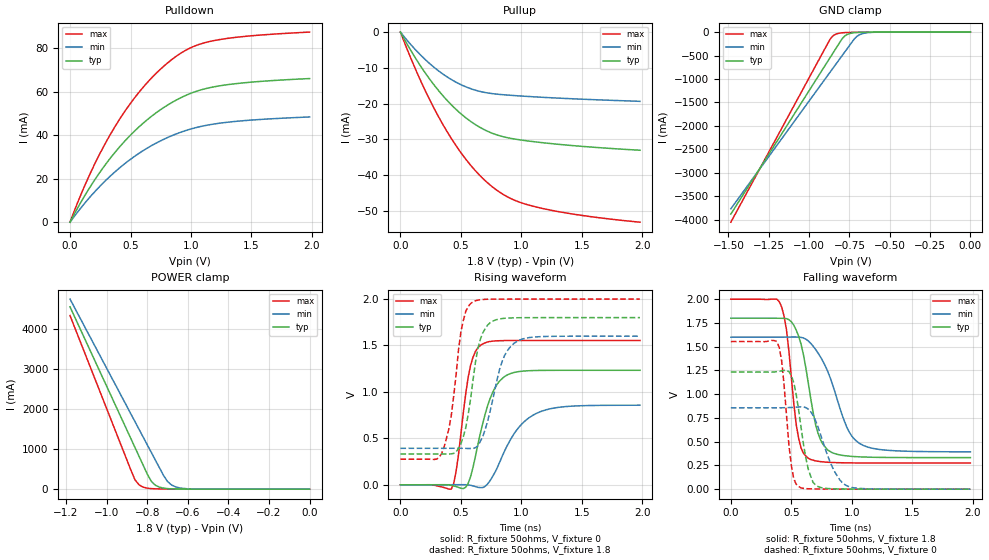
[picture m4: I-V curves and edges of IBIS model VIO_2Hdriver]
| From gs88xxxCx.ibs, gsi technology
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|  signals   DQA1-DQA9, DQB1-DQB9, DQC1-DQC9, DQD1-DQD9
[Model]   VIO_2Hdriver
Model_type   I/O
Polarity   Non-Inverting
Vinl  =   0.80v
Vinh  =   1.20v
Vmeas =   0.90v
Cref  =   0.0pF
Rref  =   50
Vref  =   0.90v
|  variable   typ   min   max
C_comp   3.0pF   2.5pF   3.5pF
|  variable   typ   min   max
[Temperature Range]   50   0   100
|  variable   typ   min   max
[Voltage Range]   1.8   1.6   2.0
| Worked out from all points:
|   slope of the pulldown table from 0 to 0.27 V, typ, clamps not added: 10.9 ohm
|   slope of the pullup table from 0 to 0.27 V, typ, clamps not added: 18.7 ohm
|   GND clamp passes 1 mA (typ) near -0.61 V on its own axis
|   POWER clamp passes 1 mA (typ) near -0.59 V on its own axis
|   rising waveform, R_fixture 50ohms, V_fixture 0: 20-80 % time 150ps typ, 233ps min, 94.8ps max; typ from 0 V to 1.23 V
|   rising waveform, R_fixture 50ohms, V_fixture 1.8: 20-80 % time 106ps typ, 141ps min, 98.2ps max; typ from 0.332 V to 1.8 V
|   falling waveform, R_fixture 50ohms, V_fixture 1.8: 20-80 % time 128ps typ, 210ps min, 86.5ps max; typ from 1.8 V to 0.332 V
|   falling waveform, R_fixture 50ohms, V_fixture 0: 20-80 % time 92.3ps typ, 153ps min, 65.9ps max; typ from 1.23 V to 0 V
[Pulldown]
| voltage   typ   min   max
0V        -286.4pA   -891.3pA   -166.8pA
80mV      8.2mA      5.874mA    11.32mA
180mV     17.4mA     12.49mA    23.94mA
280mV     25.51mA    18.36mA    35mA
380mV     32.65mA    23.54mA    44.68mA
480mV     38.89mA    28.08mA    53.1mA
600mV     45.29mA    32.74mA    61.72mA
820mV     54.3mA     39.26mA    73.82mA
1V        59.29mA    42.86mA    80.26mA
1.18V     62.12mA    45.04mA    83.37mA
1.48V     64.3mA     46.86mA    85.59mA
1.98V     66.03mA    48.39mA    87.39mA
[Pullup]
| voltage (VDDQ-Vout)   typ   min   max
0V        191.8pA    794.2pA    89.01pA
80mV      -4.802mA   -3.277mA   -6.819mA
180mV     -10.18mA   -6.867mA   -14.56mA
280mV     -14.87mA   -9.905mA   -21.45mA
380mV     -18.89mA   -12.4mA    -27.52mA
560mV     -24.48mA   -15.57mA   -36.39mA
660mV     -26.69mA   -16.61mA   -40.22mA
760mV     -28.3mA    -17.21mA   -43.28mA
920mV     -29.76mA   -17.7mA    -46.67mA
1.12V     -30.72mA   -18.13mA   -48.9mA
1.48V     -31.9mA    -18.73mA   -51.17mA
1.98V     -33.04mA   -19.37mA   -53.16mA
[GND Clamp]
| voltage   typ   min   max
-1.485V   -3.884A    -3.771A    -4.056A
-885mV    -626.9mA   -926.9mA   -247.2mA
-870mV    -545.6mA   -856mA     -153.5mA
-855mV    -464.4mA   -785mA     -89.11mA
-825mV    -301.9mA   -643.2mA   -32.88mA
-795mV    -141.5mA   -501.4mA   -15.38mA
-780mV    -86.61mA   -430.5mA   -11.65mA
-750mV    -32.85mA   -288.8mA   -7.734mA
-705mV    -8.727mA   -95.28mA   -4.834mA
-660mV    -2.907mA   -24.97mA   -2.925mA
-555mV    -316.7uA   -1.176mA   -484.9uA
0V        -278.2pA   -874.6pA   -161.2pA
[POWER Clamp]
| voltage (VDDQ-Vout)   typ   min   max
-1.18V    4.545A     4.74A      4.328A
-880mV    1.258A     1.875A     474.1mA
-860mV    1.039A     1.684A     234.3mA
-840mV    820.4mA    1.493A     107.4mA
-820mV    601.5mA    1.302A     50.64mA
-780mV    197.3mA    920.5mA    14.28mA
-760mV    99.71mA    729.7mA    9.034mA
-720mV    26.23mA    348.2mA    4.898mA
-700mV    13.96mA    192.6mA    3.916mA
-660mV    4.495mA    57.55mA    2.579mA
-560mV    510.5uA    2.941mA    648.3uA
0V        209pA      794.1pA    88.9pA
[Ramp]
| voltage   typ   min   max
dV/dt_r   1.16/125p   1.0/182p   1.35/88p
dV/dt_f   1.25/134p   1.12/205p   1.40/91p
R_load  =   50ohms
[Rising Waveform]
C_fixture =   0.0pF
R_fixture =   50ohms
V_fixture =   0
| Time   V(typ)   V(min)   V(max)
0s        2.247nV    9.209nV    987.5pV
420ps     -6.194mV   384.6uV    -47.41mV
460ps     -19.49mV   604.6uV    143.7mV
540ps     -26.68mV   586.1uV    982.9mV
580ps     87.5mV     -5.732mV   1.287V
680ps     657.7mV    -30.89mV   1.517V
820ps     1.117V     242.7mV    1.551V
960ps     1.215V     587.8mV    1.554V
1.1ns     1.23V      752.8mV    1.554V
1.98ns    1.233V     856.6mV    1.554V
[Rising Waveform]
C_fixture =   0.0pF
R_fixture =   50ohms
V_fixture =   1.8
V_fixture_min =  1.6
V_fixture_max =  2.0
| Time   V(typ)   V(min)   V(max)
0s        332.2mV    392.6mV    275.1mV
340ps     331.8mV    392.6mV    333.7mV
420ps     333.1mV    393mV      742.8mV
500ps     441mV      392.8mV    1.65V
600ps     1.129V     390.8mV    1.971V
640ps     1.467V     418.5mV    1.988V
720ps     1.72V      681mV      1.998V
840ps     1.79V      1.325V     2V
940ps     1.798V     1.525V     2V
1.98ns    1.8V       1.6V       2V
[Falling Waveform]
C_fixture =   0.0pF
R_fixture =   50ohms
V_fixture =   1.8
V_fixture_min =  1.6
V_fixture_max =  2.0
| Time   V(typ)   V(min)   V(max)
0s        1.8V       1.6V       2V
400ps     1.799V     1.6V       1.974V
460ps     1.795V     1.601V     1.678V
560ps     1.61V      1.601V     537.2mV
640ps     1.119V     1.561V     325.2mV
700ps     681.9mV    1.472V     297.8mV
760ps     474.9mV    1.349V     287.5mV
960ps     349.8mV    647.1mV    277mV
1.06ns    340.5mV    484.6mV    275.9mV
1.98ns    332.3mV    393.1mV    275.2mV
[Falling Waveform]
C_fixture =   0.0pF
R_fixture =   50ohms
V_fixture =   0
| Time   V(typ)   V(min)   V(max)
0s        1.233V     856.8mV    1.554V
380ps     1.237V     856.5mV    1.555V
420ps     1.245V     856.9mV    1.351V
500ps     1.197V     860.2mV    249.5mV
560ps     836.2mV    864.7mV    28.86mV
640ps     209.9mV    842.5mV    4.275mV
720ps     27.94mV    656.4mV    1.771mV
840ps     4.149mV    229.6mV    578.1uV
960ps     1.333mV    34.72mV    183.2uV
1.98ns    1.683uV    20.76uV    403.3nV
